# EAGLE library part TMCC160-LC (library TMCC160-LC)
TMCC160 motionCookiemicrosystem with 3-Phase BLDC/PMSM gate driver for up to 24V and 1A gate current with CAN, Hall, RS485, SPI, UART; LGA51
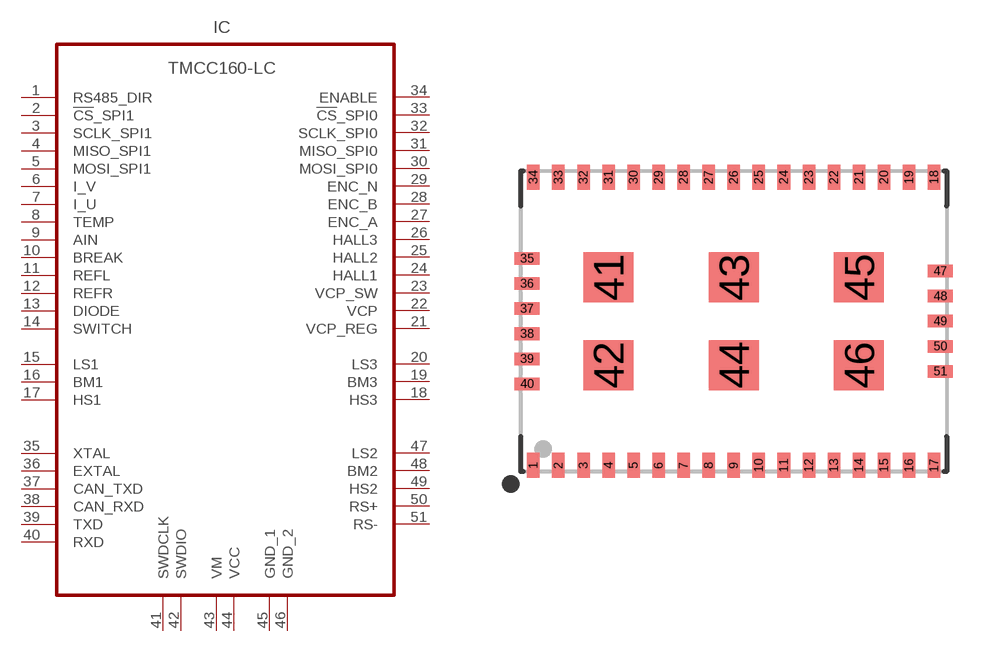
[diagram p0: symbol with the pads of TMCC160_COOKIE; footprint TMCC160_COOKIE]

Designator prefix IC

## TMCC160-LC (DATASHEET: http://www_trinamic_com/_scripts/download_php?file=_articles%2Fproducts%2Fmotioncookies%2Ftmcc160%2F_datasheet%2FTMCC160_datasheet_pdf; DESCRIPTION: TMCC160 motionCookiemicrosystem with 3-Phase BLDC/PMSM gate driver for up to 24V and 1A gate current with CAN, Hall, RS485, SPI, UART; LGA51; GEOMETRY_HEIGHT: 1,4mm; MANUFACTURER: TRINAMIC; ORDERCODE-MANU1: TMCC160-LC; VALUE: TMCC160-LC)  [TMCC160_COOKIE]
1  RS485_DIR
2  !CS!_SPI1  out
3  SCLK_SPI1  out
4  MISO_SPI1
5  MOSI_SPI1
6  I_V
7  I_U
8  TEMP
9  AIN
10  BREAK
11  REFL
12  REFR
13  DIODE
14  SWITCH
15  LS1  out
16  BM1
17  HS1  out
18  HS3  out
19  BM3
20  LS3  out
21  VCP_REG  pwr
22  VCP  pwr
23  VCP_SW  pwr
24  HALL1
25  HALL2
26  HALL3
27  ENC_A
28  ENC_B
29  ENC_N
30  MOSI_SPI0
31  MISO_SPI0
32  SCLK_SPI0  out
33  !CS!_SPI0  out
34  ENABLE  in
35  XTAL
36  EXTAL
37  CAN_TXD  out
38  CAN_RXD  in
39  TXD  out
40  RXD  in
41  SWDCLK
42  SWDIO
43  VM  out
44  VCC  out
45  GND_1  pwr
46  GND_2  pwr
47  LS2  out
48  BM2
49  HS2  out
50  RS+
51  RS-

## Footprint TMCC160_COOKIE (pad centres in mm)
smd 0.5 x 1: 1 -8,-5.75; 2 -7,-5.75; 3 -6,-5.75; 4 -5,-5.75; 5 -4,-5.75; 6 -3,-5.75; 7 -2,-5.75; 8 -1,-5.75; 9 0,-5.75; 10 1,-5.75; 11 2,-5.75; 12 3,-5.75; 13 4,-5.75; 14 5,-5.75; 15 6,-5.75; 16 7,-5.75; 17 8,-5.75; 18 8,5.75; 19 7,5.75; 20 6,5.75; 21 5,5.75; 22 4,5.75; 23 3,5.75; 24 2,5.75; 25 1,5.75; 26 0,5.75; 27 -1,5.75; 28 -2,5.75; 29 -3,5.75; 30 -4,5.75; 31 -5,5.75; 32 -6,5.75; 33 -7,5.75; 34 -8,5.75
smd 1 x 0.5: 35 -8.25,2.5; 36 -8.25,1.5; 37 -8.25,0.5; 38 -8.25,-0.5; 39 -8.25,-1.5; 40 -8.25,-2.5; 47 8.25,2; 48 8.25,1; 49 8.25,0; 50 8.25,-1; 51 8.25,-2
smd 2 x 2: 41 -5,1.75; 42 -5,-1.75; 43 0,1.75; 44 0,-1.75; 45 5,1.75; 46 5,-1.75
